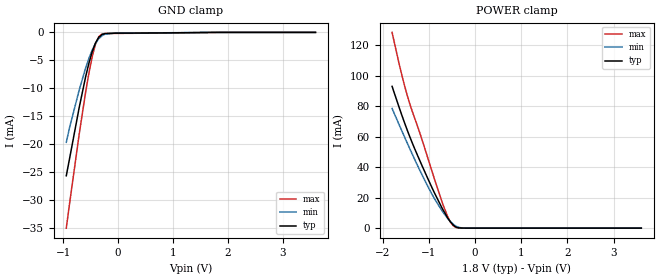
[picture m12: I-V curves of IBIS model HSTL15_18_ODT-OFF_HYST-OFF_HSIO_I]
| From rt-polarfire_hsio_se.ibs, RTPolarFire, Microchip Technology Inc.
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|   HSTL15_18_ODT-OFF_HYST-OFF_HSIO_I
[Model]   HSTL15_18_ODT-OFF_HYST-OFF_HSIO_I
Model_type  Input
Vinl =   0.65
Vinh =   0.85
|   typ   min   max
C_comp_pullup   1.335e-12   1.335e-12   1.380e-12
C_comp_pulldown  1.335e-12   1.335e-12   1.380e-12
[Temperature Range]   25   125   -55
[Voltage Range]   1.8   1.71   1.89
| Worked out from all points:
|   GND clamp passes 1 mA (typ) near -0.36 V on its own axis
|   POWER clamp passes 1 mA (typ) near -0.43 V on its own axis
[GND Clamp]
| Voltage   I(typ)   I(min)   I(max)
-945mV    -25.65mA   -19.67mA   -35.01mA
-885.9mV  -22.62mA   -17.05mA   -30.68mA
-708.7mV  -13.41mA   -10.28mA   -18.15mA
-590.6mV  -7.869mA   -6.332mA   -10.59mA
-531.6mV  -5.486mA   -4.626mA   -7.251mA
-472.5mV  -3.472mA   -3.165mA   -4.371mA
-413.4mV  -1.919mA   -1.995mA   -2.136mA
-354.4mV  -899.9uA   -1.144mA   -780.2uA
-295.3mV  -390.4uA   -603.1uA   -297.1uA
-236.2mV  -212uA     -316.1uA   -206.4uA
-59.06mV  -146.2uA   -127.5uA   -182.2uA
3.6V      0A         0A         0A
[POWER Clamp]
| Voltage   I(typ)   I(min)   I(max)
-1.8V     93.12mA    78.59mA    128.6mA
-1.595V   74.67mA    64.28mA    101.2mA
-1.417V   60.1mA     52.23mA    81.72mA
-1.181V   43.09mA    36.85mA    60.84mA
-1.004V   31.09mA    26.15mA    43.96mA
-708.7mV  12.66mA    10.92mA    16.36mA
-590.6mV  6.469mA    6.137mA    7.226mA
-531.6mV  3.923mA    4.132mA    3.797mA
-472.5mV  1.944mA    2.471mA    1.511mA
-354.4mV  179.4uA    509.1uA    86.53uA
-236.2mV  27.5uA     61.89uA    29.14uA
3.6V      0A         0A         0A
